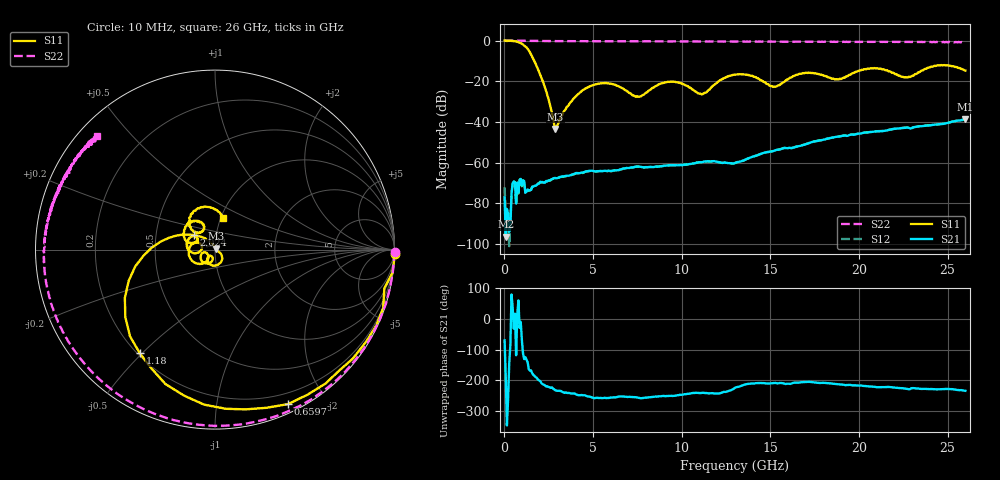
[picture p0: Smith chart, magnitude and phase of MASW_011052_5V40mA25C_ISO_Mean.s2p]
! MA-COM, USA
! Part Number: MASW-011052
! Data: 29-03-2013
! Bias Condition:
!  Isolation in OFF stage Antenna (1) to RFin (2)
!  Forward Bias (series Diode and Shunt Diode) I = 40 mA
!  Reverse Bias Voltage V = -5V
!  Temp: 25C
!  VAR RecID: Mean
# HZ S DB R 50
! F n11x n11y n21x n21y n12x n12y n22x n22y
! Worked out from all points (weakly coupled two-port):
!   401 points, 10 MHz to 26 GHz, reference 50 ohm
!   highest |S21| = -38.79 dB at 26 GHz (marker M1); lowest = -96.5 dB at 74.97 MHz (marker M2)
!   lowest |S11| = -43.5 dB at 2.869 GHz (marker M3), VSWR 1.01, Z = 50.5 + j0.453 ohm
!   |S11| at or under -10 dB: 1.684 GHz to end of sweep
!   |S22| runs from -0.9 to 0.0 dB; largest |S21 - S12| = 0.00034
!   S11 on the Smith chart (normalised r, x): 10 MHz: -12, -88; 659.8 MHz: 0.09, -1.58; 1.18 GHz: 0.21, -0.49; 2.024 GHz: 0.78, +0.13; 26 GHz: 1.02, +0.37
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1e7  0.03 -1.3  -77.06 -69.9  -72.18 177.3  0.00 -0.8
7.4975e7  -0.03 -7.5  -96.47 168.7  -86.50 124.3  -0.01 -6.5
2.0493e8  -0.07 -19.2  -85.04 94.9  -89.18 84.4  -0.01 -17.5
4.6483e8  -0.30 -44.1  -70.16 37.9  -70.38 39.5  -0.05 -38.6
6.5975e8  -0.43 -64.7  -80.16 -118.7  -80.44 -117.0  -0.07 -53.0
9.8463e8  -1.60 -102.0  -71.33 -69.7  -71.63 -71.0  -0.12 -73.7
1.1796e9  -2.93 -126.0  -74.80 -125.3  -74.85 -125.3  -0.15 -84.1
1.5694e9  -7.97 -175.2  -71.94 -178.0  -71.81 -179.1  -0.20 -101.2
2.0242e9  -16.98 145.2  -69.49 156.3  -69.40 155.7  -0.24 -116.0
2.8689e9  -43.50 42.2  -67.57 126.7  -67.59 128.3  -0.29 -134.6
4.3633e9  -24.79 -46.1  -64.95 110.9  -65.06 110.6  -0.32 -153.4
5.7928e9  -20.97 -100.9  -64.10 101.2  -64.26 101.5  -0.35 -164.3
7.5471e9  -27.60 -117.5  -61.89 102.0  -62.05 102.5  -0.39 -173.6
8.7167e9  -21.51 -114.5  -61.93 106.9  -61.88 106.8  -0.41 -178.2
9.8212e9  -20.69 -150.8  -61.29 110.1  -61.44 110.7  -0.43 177.5
1.1121e10  -26.47 -146.9  -59.82 118.0  -59.71 118.3  -0.49 173.2
1.3005e10  -16.77 -158.3  -60.20 134.7  -60.23 135.1  -0.51 167.8
1.5214e10  -22.61 173.3  -54.18 150.3  -54.17 151.0  -0.56 162.7
1.7358e10  -15.93 159.5  -49.85 152.7  -49.86 153.8  -0.58 157.6
1.8723e10  -18.97 153.2  -47.32 146.8  -47.32 147.8  -0.65 154.6
2.1712e10  -15.22 119.5  -43.92 137.2  -43.82 138.4  -0.67 147.8
2.6e10  -14.79 76.6  -38.79 124.6  -38.73 126.3  -0.77 136.0
